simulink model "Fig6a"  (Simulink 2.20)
settings: Solver=ode45  StartTime=0.0  StopTime=10.0  RelTol=1e-3  AbsTol=1e-6
libraries: simulink x1

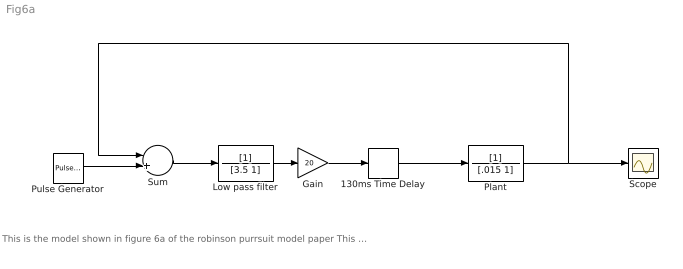
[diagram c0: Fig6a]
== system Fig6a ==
  note: This is the model shown in figure 6a of the robinson purrsuit model paper This is the simplest possible model, the most interesting thing is to tweak the first low-pass filter to examine how that effects the oscillatory stability of the model Actually, that's the only parameter to tweak because you need a total pursuit gain of .95 which requires a gain of 20 (Gain/1+gain).
  130ms Time Delay : TransportDelay  DelayTime=.13  InitialInput=0  BufferSize=1024
  Gain : Gain  Gain=20
  Low pass filter : TransferFcn  Numerator=[1]  Denominator=[3.5 1]
  Plant : TransferFcn  Numerator=[1]  Denominator=[.015 1]
  Pulse Generator : simulink/Sources/Pulse Generator  period=100  duty=50  amplitude=20  start=0
  Scope : Scope
  Sum : Sum  Inputs=-+
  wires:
  Pulse Generator/1 -> Sum/2
  Gain/1 -> 130ms Time Delay/1
  130ms Time Delay/1 -> Plant/1
  Low pass filter/1 -> Gain/1
  Sum/1 -> Low pass filter/1
  Plant/1 -> Scope/1, Sum/1
